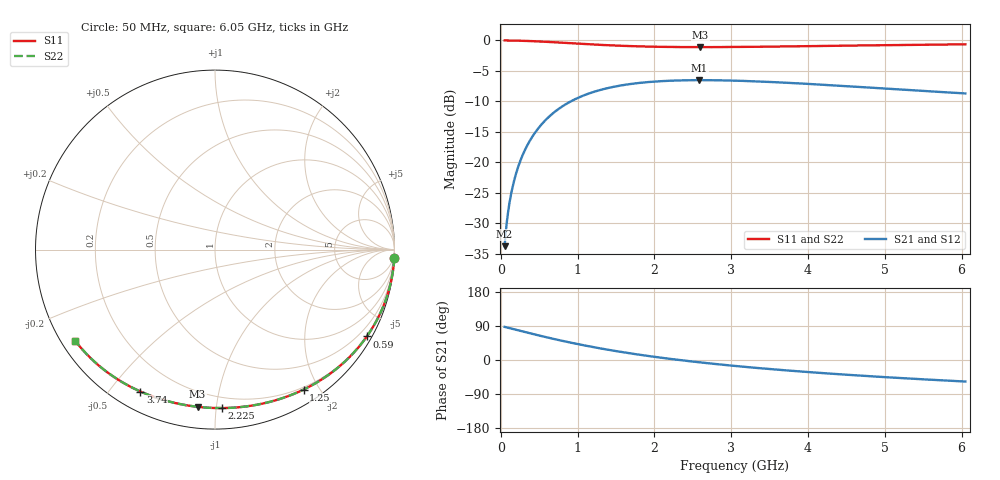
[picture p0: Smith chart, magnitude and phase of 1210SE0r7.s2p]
! AVX Thin Film Operation		Date: August 2001
! Description: Accu-P® Series, Thin Film, SMD, RF Capacitor
! Part Number: 12101J0R7ABT
! 50 MHz  -  6.05 GHz
! Serial Measurements
# mhz S db R 50
!	S11		S21		S12		S22
!	dB	Phase	dB	Phase	dB	Phase	dB	Phase
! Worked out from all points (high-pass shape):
!   401 points, 50 MHz to 6.05 GHz, reference 50 ohm
!   highest |S21| = -6.52 dB at 2.585 GHz (marker M1); lowest = -33.8 dB at 50 MHz (marker M2)
!   |S21| within 3 dB of the highest: 989.2 MHz to end of sweep
!   lowest |S11| = -1.1 dB at 2.6 GHz (marker M3), VSWR 15.86, Z = 5.66 - j44.4 ohm
!   |S11| at or under -10 dB: nowhere
!   |S22| runs from -1.1 to 0.0 dB; largest |S21 - S12| = 5.1e-05
!   S11 on the Smith chart (normalised r, x): 50 MHz: 0, -44; 590 MHz: 0.19, -3.75; 1.25 GHz: 0.17, -1.80; 2.225 GHz: 0.13, -1.04; 3.74 GHz: 0.08, -0.60; 6.05 GHz: 0.04, -0.30
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50  -0.00 -2.6  -33.78 87.4  -33.78 87.4  -0.00 -2.6
65  -0.00 -3.4  -31.51 86.6  -31.51 86.6  -0.00 -3.4
110  -0.01 -5.7  -26.95 84.3  -26.95 84.3  -0.01 -5.7
140  -0.01 -7.3  -24.87 82.7  -24.87 82.7  -0.01 -7.3
185  -0.03 -9.6  -22.48 80.4  -22.48 80.4  -0.03 -9.6
230  -0.04 -11.9  -20.62 78.1  -20.62 78.1  -0.04 -11.9
305  -0.07 -15.8  -18.25 74.2  -18.25 74.2  -0.07 -15.8
380  -0.10 -19.5  -16.44 70.5  -16.44 70.5  -0.10 -19.5
590  -0.22 -29.8  -12.99 60.2  -12.99 60.2  -0.22 -29.8
800  -0.37 -39.4  -10.84 50.6  -10.84 50.6  -0.37 -39.4
1055  -0.56 -50.1  -9.16 39.9  -9.16 39.9  -0.56 -50.1
1250  -0.70 -57.6  -8.29 32.3  -8.29 32.3  -0.70 -57.7
1625  -0.90 -70.5  -7.27 19.5  -7.27 19.5  -0.90 -70.5
2060  -1.04 -83.2  -6.71 6.8  -6.71 6.8  -1.04 -83.2
2225  -1.07 -87.5  -6.61 2.5  -6.61 2.5  -1.07 -87.5
2585  -1.10 -96.0  -6.52 -6.0  -6.52 -6.0  -1.10 -96.0
2600  -1.10 -96.3  -6.52 -6.4  -6.52 -6.4  -1.10 -96.4
3050  -1.07 -105.6  -6.60 -15.7  -6.60 -15.7  -1.07 -105.7
3740  -0.98 -117.7  -6.96 -27.8  -6.96 -27.8  -0.98 -117.7
4055  -0.93 -122.6  -7.17 -32.6  -7.17 -32.6  -0.93 -122.6
5060  -0.77 -135.9  -7.94 -45.9  -7.94 -45.9  -0.77 -135.9
6050  -0.63 -146.8  -8.70 -56.9  -8.70 -56.9  -0.64 -146.8
